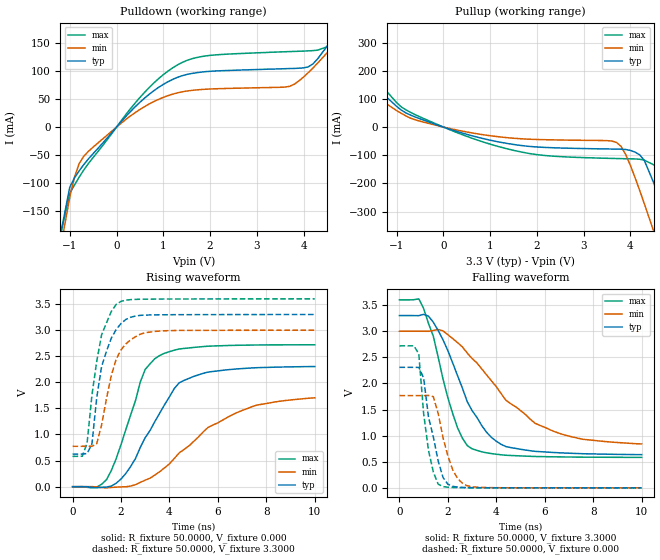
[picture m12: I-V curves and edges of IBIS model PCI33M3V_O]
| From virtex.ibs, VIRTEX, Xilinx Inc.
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|   Model PCI33M3V_O
[Model]   PCI33M3V_O
Model_type   Output
Polarity   Non-Inverting
| Vmeas depends on rising or falling edge, select one of the following:
| For rising edge:
|Vmeas =   0.940V
| For falling edge:
|Vmeas =   2.00V
Cref =  10.0000pF
Rref =  25.0000
| Vref depends on rising or falling edge, select one of the following:
| For rising edge:
|Vref =   0.00V
| For falling edge:
|Vref =   3.30V
C_comp   6.5000pF   5.0000pF   8.0000pF
[Temperature Range]   27.0000   100.0000   0.000
[Voltage Range]   3.3000V   3.0000V   3.6000V
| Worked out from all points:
|   slope of the pulldown table from 0 to 0.495 V, typ, clamps not added: 11.3 ohm
|   slope of the pullup table from 0 to 0.495 V, typ, clamps not added: 19.4 ohm
|   rising waveform, R_fixture 50.0000, V_fixture 0.000: 20-80 % time 1.66ns typ, 2.79ns min, 1.13ns max; typ from 0 V to 2.3 V
|   rising waveform, R_fixture 50.0000, V_fixture 3.3000: 20-80 % time 658ps typ, 711ps min, 598ps max; typ from 0.625 V to 3.3 V
|   falling waveform, R_fixture 50.0000, V_fixture 3.3000: 20-80 % time 1.57ns typ, 2.68ns min, 1.05ns max; typ from 3.3 V to 0.636 V
|   falling waveform, R_fixture 50.0000, V_fixture 0.000: 20-80 % time 564ps typ, 590ps min, 415ps max; typ from 2.31 V to 0 V
[Pulldown]
| voltage   I(typ)   I(min)   I(max)
-3.3V     -1.282A    -1.27A     -1.284A
-1.5V     -320.5mA   -355mA     -308.6mA
-1V       -107.1mA   -125mA     -118mA
-800mV    -78.31mA   -65.17mA   -89.55mA
-600mV    -56.71mA   -43.28mA   -64.84mA
600mV     51.72mA    36.54mA    62.03mA
1.5V      93.89mA    64.31mA    118.9mA
3.7V      104.5mA    72.65mA    134.8mA
4.2V      112.6mA    105.3mA    136.5mA
4.5V      143.9mA    132.2mA    143.3mA
4.9V      194.6mA    171.6mA    196.4mA
6.6V      424.6mA    347.8mA    474.2mA
[Pullup]
| voltage   I(typ)   I(min)   I(max)
-3.3V     423.8mA    325.6mA    510mA
-2.9V     366mA      280.2mA    440.1mA
-2.3V     275.3mA    208.6mA    331.8mA
-600mV    35.56mA    25.59mA    43.66mA
1.6V      -64.04mA   -40.84mA   -86.17mA
3.7V      -78.19mA   -54.2mA    -111.6mA
3.9V      -79.49mA   -97.57mA   -112.4mA
4.2V      -98.59mA   -225.3mA   -114.1mA
4.5V      -198.1mA   -370.5mA   -134mA
4.9V      -397.4mA   -571.2mA   -249.8mA
5.1V      -502.7mA   -672.9mA   -347.5mA
6.6V      -1.313A    -1.445A    -1.162A
[Ramp]
| variable   typ   min   max
dV/dt_r   1.3812/1.6793n   1.0212/2.7825n   1.6314/1.1743n
dV/dt_f   1.5983/1.5591n   1.2952/2.6998n   1.8097/1.0214n
R_load = 50.0000
[Rising Waveform]
R_fixture = 50.0000
V_fixture = 0.000
| time   V(typ)   V(min)   V(max)
0s        0V         0V         0V
1ns       -21.37mV   -4.968mV   -6.56mV
1.4ns     -7.112mV   -22.34mV   133.5mV
2.2ns     254.2mV    -1.69mV    1.095V
3ns       940mV      124.7mV    2.247V
3.6ns     1.411V     288.9mV    2.514V
4.4ns     1.989V     646.6mV    2.638V
5.4ns     2.173V     1.053V     2.685V
7.6ns     2.28V      1.562V     2.715V
10ns      2.302V     1.702V     2.719V
[Rising Waveform]
R_fixture = 50.0000
V_fixture = 3.3000
V_fixture_min = 3.0000
V_fixture_max = 3.6000
| time   V(typ)   V(min)   V(max)
0s        625mV      774mV      581.5mV
400ps     625.4mV    774.1mV    582.9mV
600ps     634.4mV    774.5mV    833.4mV
800ps     817.2mV    774.3mV    1.753V
1ns       1.714V     826.4mV    2.411V
1.2ns     2.304V     1.185V     2.911V
1.8ns     3.01V      2.442V     3.491V
2.2ns     3.204V     2.736V     3.575V
3ns       3.288V     2.95V      3.593V
10ns      3.299V     2.998V     3.599V
[Falling Waveform]
R_fixture = 50.0000
V_fixture = 3.3000
V_fixture_min = 3.0000
V_fixture_max = 3.6000
| time   V(typ)   V(min)   V(max)
0s        3.3V       3V         3.6V
800ps     3.298V     3V         3.62V
1ns       3.324V     3V         3.434V
1.6ns     3.013V     3.033V     2.502V
2.4ns     2.148V     2.782V     1.149V
3ns       1.48V      2.477V     747.4mV
4.2ns     833.1mV    1.804V     633.1mV
5.6ns     699.5mV    1.237V     600.9mV
7.6ns     653.4mV    929mV      588.1mV
10ns      636.2mV    841.4mV    583.8mV
[Falling Waveform]
R_fixture = 50.0000
V_fixture = 0.000
| time   V(typ)   V(min)   V(max)
0s        2.309V     1.768V     2.72V
800ps     2.308V     1.768V     2.564V
1ns       2.106V     1.768V     1.42V
1.2ns     1.355V     1.77V      715.4mV
1.4ns     974mV      1.746V     303.7mV
1.6ns     513.3mV    1.423V     71.11mV
1.8ns     199.7mV    962mV      24.36mV
2.2ns     29.02mV    346.4mV    7.88mV
2.8ns     5.398mV    39.2mV     3.043mV
10ns      293.2uV    457.1uV    223.9uV
